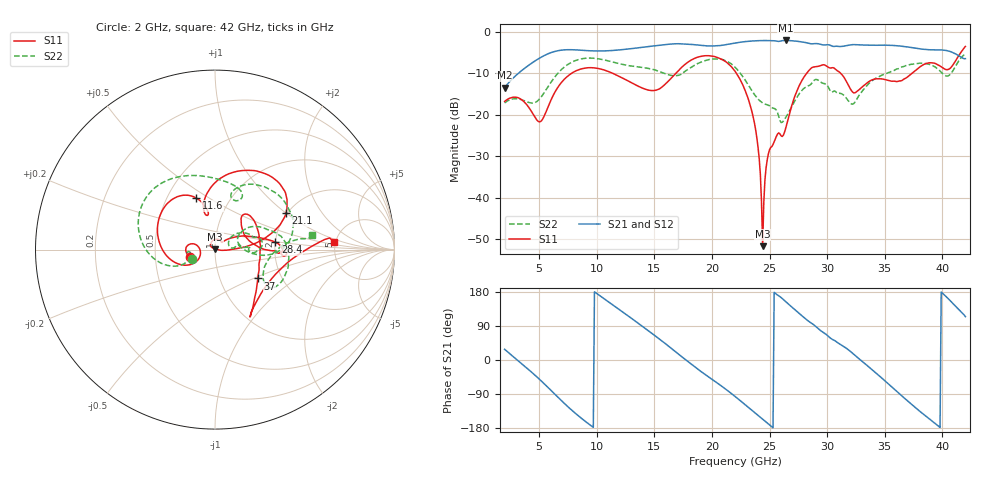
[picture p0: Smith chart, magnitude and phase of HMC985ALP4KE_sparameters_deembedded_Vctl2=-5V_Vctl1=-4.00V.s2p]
!s2p File: Measurements: S11, S21, S12, S22
# GHz S dB R 50.0
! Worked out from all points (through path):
!   401 points, 2 GHz to 42 GHz, reference 50 ohm
!   highest |S21| = -2.10 dB at 26.4 GHz (marker M1); lowest = -13.5 dB at 2 GHz (marker M2)
!   lowest |S11| = -51.7 dB at 24.4 GHz (marker M3), VSWR 1.01, Z = 50.1 + j0.253 ohm
!   |S11| at or under -10 dB: start of sweep to 7.821 GHz; 22.12 GHz to 28.22 GHz (6.106 GHz wide, 24.3 % of centre); 31.17 GHz to 37.37 GHz (6.196 GHz wide, 18.1 % of centre)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
!   |S22| runs from -21.9 to -5.3 dB; largest |S21 - S12| = 0.00083
!   S11 on the Smith chart (normalised r, x): 2 GHz: 0.75, -0.07; 11.6 GHz: 0.70, +0.44; 21.1 GHz: 1.97, +1.00; 28.4 GHz: 2.00, +0.19; 37 GHz: 1.51, -0.53; 42 GHz: 4.84, +0.77
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2  -16.77 -162.4  -13.48 28.3  -13.48 28.3  -17.15 -156.8
5  -21.69 -174.2  -6.41 -50.1  -6.41 -50.1  -16.29 -160.2
6.3  -14.90 -151.2  -4.79 -88.4  -4.79 -88.4  -11.10 -161.6
8.7  -8.92 150.0  -4.46 -154.6  -4.46 -154.6  -6.51 151.3
11.6  -10.29 110.0  -4.46 140.8  -4.47 140.8  -7.44 103.6
13.6  -13.12 100.8  -3.87 96.9  -3.87 97.0  -8.48 76.1
15.4  -13.81 105.4  -3.27 56.1  -3.27 56.1  -9.54 62.8
17.9  -7.35 79.7  -2.97 -3.9  -2.98 -3.9  -9.09 72.1
21.1  -7.05 27.1  -3.16 -74.8  -3.16 -74.7  -6.90 15.9
22  -9.50 16.6  -2.73 -96.0  -2.73 -96.0  -8.52 0.6
23.6  -20.82 0.3  -2.20 -135.8  -2.20 -135.8  -14.76 -3.5
24.4  -51.66 75.2  -2.11 -156.0  -2.12 -155.9  -17.14 7.7
25  -28.40 132.2  -2.15 -171.3  -2.15 -171.2  -17.82 11.0
26.4  -23.27 43.8  -2.10 154.0  -2.10 154.1  -20.68 32.8
28.4  -9.39 7.1  -2.78 102.1  -2.78 102.1  -12.99 18.2
28.7  -8.60 1.9  -2.91 95.9  -2.92 95.9  -12.24 16.5
30.7  -8.99 -3.3  -3.50 50.4  -3.50 50.4  -14.34 2.5
32.5  -14.56 34.2  -3.12 10.0  -3.12 10.0  -16.61 29.4
35.4  -11.75 18.3  -3.25 -65.4  -3.25 -65.3  -9.78 19.2
37  -10.83 -33.9  -3.68 -108.4  -3.68 -108.4  -8.04 4.8
39.8  -8.25 -56.4  -4.38 -178.0  -4.38 -178.0  -9.45 -34.4
42  -3.54 3.8  -6.48 114.5  -6.48 114.5  -5.28 8.5
